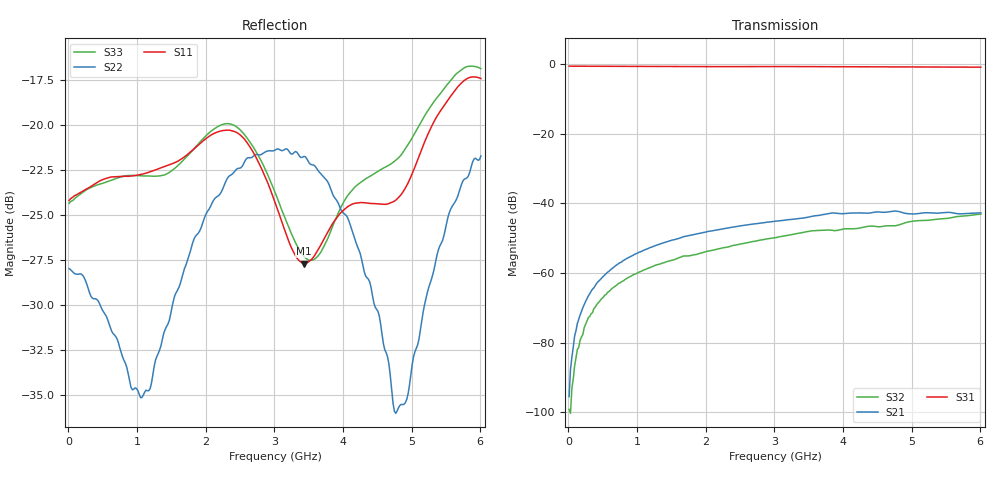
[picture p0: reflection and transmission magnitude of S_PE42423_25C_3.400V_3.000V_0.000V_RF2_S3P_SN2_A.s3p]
! Device ID: PE42423_Char_Units
! Serial: 2
! Insertion: A
! Temp: 25C
! VDD: 3.400
! Control_Hi: 3.000
! Control_Lo: 0.000
! Logic State: RF2
! ThroughPath: 3-1
! Port 1: RFC
! Port 2: RF1
! Port 3: RF2
! V1 = 3.00
! V2 = 3.00
! V3 = 0.00
! IDD: 1.359909e-04
! FILE NAME
! DATE 07-24-2013 19:16:06
! CORRECTED  DATA
#  Hz  S  RI  R  50
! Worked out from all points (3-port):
!   301 points, 10 MHz to 6.01 GHz, reference 50 ohm
!   strongest paths, dB at 10 MHz, 1.51 GHz, 3.01 GHz, 4.51 GHz, 6.01 GHz:
!     S31: -0.6, -0.7, -0.7, -0.8, -0.9
!     S21: -95.5, -50.6, -45.1, -42.5, -42.7
!     S32: -99.2, -56.3, -49.9, -46.7, -43.1
!   lowest |S11| = -27.7 dB at 3.43 GHz (marker M1), VSWR 1.09, Z = 53.3 - j2.73 ohm
!   |S11| at or under -10 dB: start of sweep to end of sweep
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1e7  0.0618 -0.000139  -5.32e-06 -4.89e-06  0.9299 -0.00288
     1.27e-05 -1.11e-05  -0.0399 0.000206  -4.92e-06 -7.08e-06
     0.9305 -0.00292  2.69e-06 -1.07e-05  0.0606 -0.000555
1.7e8  0.0649 -0.0022  -4.25e-05 0.000249  0.9279 -0.0407
       -3.57e-05 0.000246  -0.0386 0.00188  -4.21e-05 9.04e-05
       0.9284 -0.0402  -5.03e-05 9.59e-05  0.0642 -0.0036
3.5e8  0.0677 -0.00707  -7.8e-05 0.000568  0.9238 -0.0821
       -8.72e-05 0.000579  -0.033 0.00203  -0.000106 0.000258
       0.9242 -0.0815  -9.31e-05 0.000252  0.0668 -0.0091
8.3e8  0.0707 -0.0141  -2.28e-05 0.00156  0.9042 -0.1898
       -2.77e-05 0.00158  -0.0207 0.00692  -0.000139 0.000798
       0.9052 -0.1895  -0.000151 0.000802  0.0707 -0.0154
1.19e9  0.0741 -0.00368  0.000177 0.0023  0.8818 -0.2681
        0.000168 0.00232  -0.00766 0.0169  -9.96e-05 0.00118
        0.8826 -0.2673  -9.89e-05 0.0012  0.0721 -0.00522
2.35e9  0.0853 0.046  0.00144 0.00426  0.7706 -0.4944
        0.00143 0.00426  -0.0078 0.072  9.15e-05 0.0024
        0.7719 -0.4943  8.16e-05 0.0024  0.092 0.0416
3.01e9  0.0598 0.0127  0.00233 0.00503  0.6835 -0.6146
        0.00234 0.00503  -0.0382 0.0763  0.000341 0.0032
        0.6842 -0.6132  0.000316 0.00319  0.0646 0.00865
3.43e9  0.0323 -0.0256  0.00283 0.00548  0.6139 -0.6815
        0.00282 0.0055  -0.0549 0.0608  0.000571 0.00382
        0.6151 -0.6808  0.000559 0.0038  0.0355 -0.0247
4.77e9  0.0347 -0.0513  0.00552 0.00543  0.3575 -0.8353
        0.0055 0.00545  -0.00632 -0.0145  0.000936 0.00474
        0.3594 -0.8354  0.000913 0.00469  0.037 -0.0709
6.01e9  0.1339 -0.0163  0.00509 0.00521  0.0929 -0.8959
        0.00507 0.00525  0.0651 0.0501  0.00125 0.00694
        0.0953 -0.8953  0.00122 0.00692  0.1372 -0.0429
